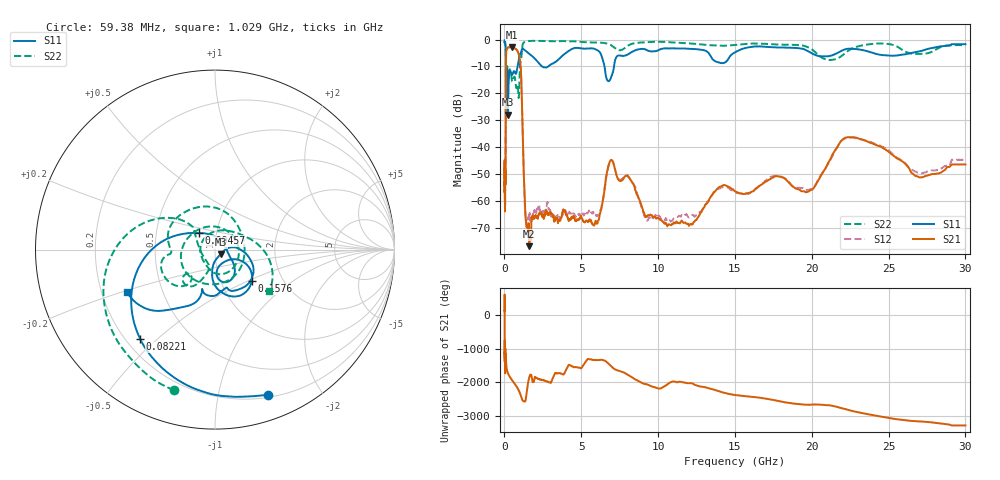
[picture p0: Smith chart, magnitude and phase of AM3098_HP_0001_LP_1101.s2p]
! Date/Time: Thu, Feb 28, 2019 8:32 AM
! Network Analyzer: Agilent Technologies E8364B Rev: A.07.50.67
! Sweep from 0.010 to 30.000 GHz, 1601 Points, Sweep Type: LOG
! Power Supply: 5.022 V, 0.002 A
# Hz S DB R 50
!freq MagS11 AngS11 MagS21 AngS21 MagS12 AngS12 MagS22 AngS22
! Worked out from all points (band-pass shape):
!   1601 points, 10 MHz to 30 GHz, reference 50 ohm
!   highest |S21| = -2.78 dB at 488.2 MHz (marker M1); lowest = -76.9 dB at 1.606 GHz (marker M2)
!   |S21| within 3 dB of the highest: 105.8 MHz to 944.5 MHz (838.7 MHz wide, 160 % of centre)
!   lowest |S11| = -27.9 dB at 232.8 MHz (marker M3), VSWR 1.08, Z = 53.1 - j2.73 ohm
!   |S11| at or under -10 dB: 91.06 MHz to 849.4 MHz (758.3 MHz wide, 161 % of centre); 2.457 GHz to 2.838 GHz (381.2 MHz wide, 14.4 % of centre); 6.514 GHz to 7.131 GHz (617.2 MHz wide, 9.05 % of centre)
!   |S22| runs from -22.5 to -0.4 dB; largest |S21 - S12| = 0.0091
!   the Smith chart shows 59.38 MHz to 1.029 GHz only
!   S11 on the Smith chart (normalised r, x): 59.38 MHz: 0.23, -1.41; 82.21 MHz: 0.26, -0.44; 94.57 MHz: 0.82, +0.16; 157.6 MHz: 1.40, -0.53; 1.029 GHz: 0.31, -0.21
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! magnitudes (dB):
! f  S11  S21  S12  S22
! 10 MHz  -0.3  -48.3  -45.9  -0.6
! 38.04 MHz  -0.5  -59.7  -61.1  -1.0
! 59.38 MHz  -1.3  -52.5  -51.1  -1.8
! 72.91 MHz  -2.1  -51.7  -50.4  -2.6
! 82.21 MHz  -3.7  -33.5  -33.5  -4.2
! 94.57 MHz  -17.8  -11.2  -11.2  -21.0
! 144.7 MHz  -14.5  -3.5  -3.4  -12.8
! 157.6 MHz  -11.4  -3.4  -3.4  -10.7
! 232.8 MHz  -27.9  -2.9  -2.9  -12.1
! 488.2 MHz  -13.1  -2.8  -2.8  -15.4
! 550.5 MHz  -12.4  -3.0  -3.0  -14.9
! 1.029 GHz  -5.3  -8.6  -8.6  -8.4
! 1.355 GHz  -4.1  -64.0  -64.8  -0.7
! 1.606 GHz  -5.2  -76.9  -65.6  -0.5
! 2.084 GHz  -7.7  -66.2  -63.9  -0.5
! 5.9 GHz  -3.5  -68.2  -65.1  -1.0
! 6.855 GHz  -15.1  -45.4  -45.4  -1.8
! 7.926 GHz  -5.8  -50.6  -50.4  -2.7
! 11.77 GHz  -3.3  -68.0  -65.2  -1.3
! 19.7 GHz  -4.1  -56.7  -56.1  -2.7
! 22.67 GHz  -3.4  -36.3  -36.5  -3.2
! 30 GHz  -1.7  -46.5  -44.7  -2.1
